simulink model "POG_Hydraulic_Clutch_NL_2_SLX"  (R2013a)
settings: Solver=ode45  StartTime=0.0  StopTime=10.0  MaxStep=0.001  RelTol=1e-3
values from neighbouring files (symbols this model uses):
  A = 5*cm^2    (= 0.0005)    [POG_Hydraulic_Clutch_NL_2_SLX_m.m]    (also in POG_Hydraulic_Clutch_SS_NL_SLX_m.m = 5*cm^2; POG_Hydraulic_Clutch_SS_SLX_m.m = 1)
  b_p = 10    [POG_Hydraulic_Clutch_NL_2_SLX_m.m]    (also in POG_Hydraulic_Clutch_SS_NL_SLX_m.m; POG_Hydraulic_Clutch_SS_SLX_m.m = 1)
  C_m = 1e-9    (= 1e-09)    [POG_Hydraulic_Clutch_NL_2_SLX_m.m]    (also in POG_Hydraulic_Clutch_SS_NL_SLX_m.m; POG_Hydraulic_Clutch_SS_SLX_m.m = 1; POG_Hydraulic_Clutch_SS_When_Cm_is_0.m = 0)
  I_0 = 0*Amp    (= 0)    [POG_Hydraulic_Clutch_NL_2_SLX_m.m]
  k1 = 150    [POG_Hydraulic_Clutch_NL_2_SLX_m.m]
  k2 = 1000    [POG_Hydraulic_Clutch_NL_2_SLX_m.m]
  K_m = P_a_t*A/(3*cm)    (= 16887.5)    [POG_Hydraulic_Clutch_NL_2_SLX_m.m]    (also in POG_Hydraulic_Clutch_SS_NL_SLX_m.m = P_a_0*A/(3*cm); POG_Hydraulic_Clutch_SS_SLX_m.m = 1; POG_Electro_Hydraulic_Pump_NL_SLX_m.m = 0.5; POG_Electro_Hydraulic_Pump_Rele_SLX_m.m = 0.5)
  K_v = (80*cm)^3/(sec*(0.2*atm))    (= 2.52652356279e-05)    [POG_Hydraulic_Clutch_NL_2_SLX_m.m]    (also in POG_Hydraulic_Clutch_SS_NL_SLX_m.m = (10*cm)^3/(sec*(0.2*atm)); POG_Hydraulic_Clutch_SS_SLX_m.m = 1)
  m_p = 300*gr    (= 0.3)    [POG_Hydraulic_Clutch_NL_2_SLX_m.m]    (also in POG_Hydraulic_Clutch_SS_NL_SLX_m.m = 300*gr; POG_Hydraulic_Clutch_SS_SLX_m.m = 1)
  P_1_0 = 0    [POG_Hydraulic_Clutch_NL_2_SLX_m.m]
  P_a_t = 10*atm    (= 1013250)    [POG_Hydraulic_Clutch_NL_2_SLX_m.m]
  Ts = Tfin/Nr_Ts_Points    (= 0.0002)    [POG_Hydraulic_Clutch_NL_2_SLX_m.m]    (also in POG_Hydraulic_Clutch_SS_NL_SLX_m.m; POG_Hydraulic_Clutch_SS_SLX_m.m = 0.005; POG_Electro_Hydraulic_Pump_NL_SLX_m.m = 0.03; POG_Electro_Hydraulic_Pump_Rele_SLX_m.m = 0.035)
  v_d_t = 0    [POG_Hydraulic_Clutch_NL_2_SLX_m.m]
  v_p_0 = 0    [POG_Hydraulic_Clutch_NL_2_SLX_m.m]
  x0 = 1.5*cm    (= 0.015)    [POG_Hydraulic_Clutch_NL_2_SLX_m.m]
  x_p_0 = 0    [POG_Hydraulic_Clutch_NL_2_SLX_m.m]
undefined symbols (not defined in the file or in its folder): sgn

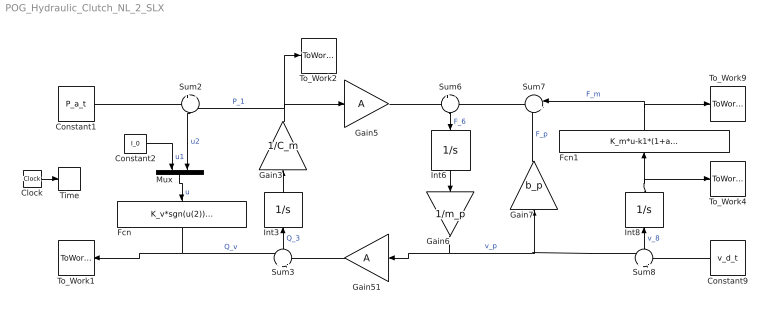
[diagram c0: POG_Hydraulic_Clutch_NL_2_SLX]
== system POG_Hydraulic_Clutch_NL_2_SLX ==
  Clock : Clock
  Constant1 : Constant  Value=P_a_t
  Constant2 : Constant  Value=I_0
  Constant9 : Constant  Value=v_d_t
  Fcn : Fcn  Expr=K_v*sgn(u(2))*sqrt(abs(u(2)))
  Fcn1 : Fcn  Expr=K_m*u-k1*(1+atan(k2*(u-x0))/(pi/2))
  Gain3 : Gain  Gain=1/C_m
  Gain5 : Gain  Gain=A
  Gain51 : Gain  Gain=A
  Gain6 : Gain  Gain=1/m_p
  Gain7 : Gain  Gain=b_p
  Int3 : Integrator  InitialCondition=P_1_0*C_m
  Int6 : Integrator  InitialCondition=v_p_0*m_p
  Int8 : Integrator  InitialCondition=x_p_0
  Mux : Mux  Inputs=2
  Sum{2..3,6,8} (4 alike) : Sum  Inputs=+|-
  Sum7 : Sum  Inputs=|++
  Time : ToWorkspace  VariableName=t  SampleTime=Ts
  To_Work1 : ToWorkspace  VariableName=Q_a_t  SampleTime=Ts
  To_Work2 : ToWorkspace  VariableName=P_1  SampleTime=Ts
  To_Work4 : ToWorkspace  VariableName=x_p  SampleTime=Ts
  To_Work9 : ToWorkspace  VariableName=F_d_t  SampleTime=Ts
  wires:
  Constant1/1 -> Sum2/1
  Gain3/1 -> To_Work2/1, Sum2/2, Gain5/1  "P_1"
  Fcn/1 -> To_Work1/1, Sum3/1  "Q_v"
  Sum2/1 -> Mux/2  "u2"
  Gain51/1 -> Sum3/2
  Sum3/1 -> Int3/1  "Q_3"
  Int3/1 -> Gain3/1
  Gain5/1 -> Sum6/1
  Gain6/1 -> Gain51/1, Gain7/1, Sum8/1  "v_p"
  Sum7/1 -> Sum6/2
  Sum6/1 -> Int6/1  "F_6"
  Int6/1 -> Gain6/1
  Fcn1/1 -> To_Work9/1, Sum7/1  "F_m"
  Gain7/1 -> Sum7/2  "F_p"
  Constant9/1 -> Sum8/2
  Sum8/1 -> Int8/1  "v_8"
  Int8/1 -> To_Work4/1, Fcn1/1
  Clock/1 -> Time/1
  Mux/1 -> Fcn/1  "u"
  Constant2/1 -> Mux/1  "u1"
